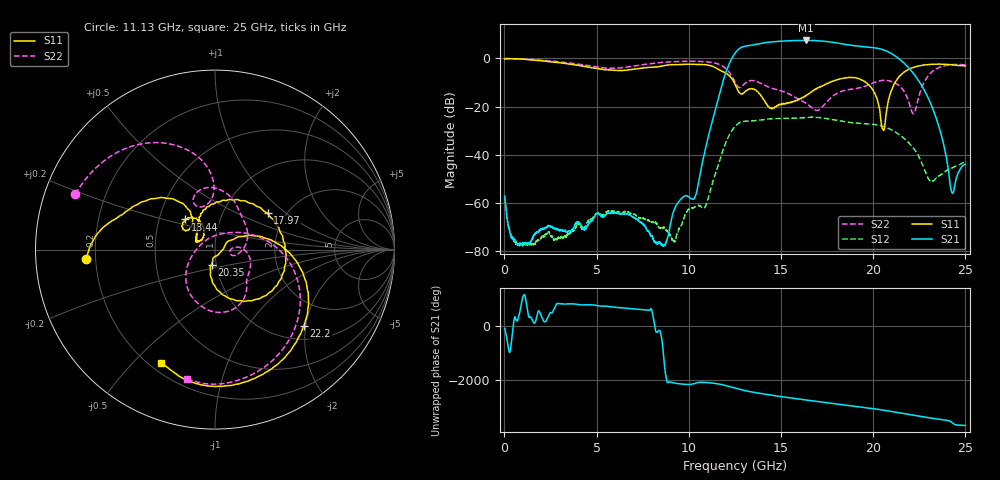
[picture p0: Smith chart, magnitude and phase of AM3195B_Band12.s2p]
!Agilent Technologies,E8364B,MY43040894,A.07.50.67
!Agilent E8364B: A.07.50.67
!Date: Wednesday, July 07, 2021 13:12:42
!Correction: S11(Full 2 Port(1,2))
!S21(Full 2 Port(1,2))
!S12(Full 2 Port(1,2))
!S22(Full 2 Port(1,2))
!S2P File: Measurements: S11, S21, S12, S22:
# Hz S  dB  R 50
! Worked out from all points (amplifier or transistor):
!   8001 points, 10 MHz to 25 GHz, reference 50 ohm
!   highest |S21| = 7.4 dB at 16.37 GHz (marker M1)
!   |S21| within 3 dB of that: 12.82 GHz to 20.05 GHz (7.233 GHz wide, 44 % of centre)
!   unconditionally stable (mu >= 1): start of sweep to end of sweep
!   at 4.174 GHz: K = 1124994.23, MAG = -63.0 dB, |S12| = -70.4 dB
!   at 12.51 GHz: K = 8.23, MAG = 3.0 dB, |S12| = -28.2 dB
!   at 25 GHz: K = 2685.67, MAG = -37.7 dB, |S12| = -43.2 dB
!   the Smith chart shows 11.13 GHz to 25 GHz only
!   S11 on the Smith chart (normalised r, x): 11.13 GHz: 0.16, -0.04; 13.44 GHz: 0.68, +0.24; 17.97 GHz: 1.62, +0.75; 20.35 GHz: 0.95, -0.16; 22.2 GHz: 1.32, -1.95; 25 GHz: 0.25, -0.60
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1e7  -0.26 -1.9  -57.06 -94.1  -57.55 83.0  -0.09 -2.8
1.918611e9  -0.92 -94.0  -71.18 127.3  -74.89 106.2  -0.70 -89.7
4.177082e9  -3.12 165.0  -69.48 53.9  -70.54 61.3  -2.58 164.4
6.594865e9  -4.90 28.7  -64.47 -68.9  -63.62 -58.0  -3.66 7.8
8.341041e9  -3.46 -62.9  -76.27 171.8  -69.73 -159.4  -1.81 -88.2
1.113055e10  -2.87 -175.9  -30.27 43.1  -55.73 -125.9  -1.54 158.3
1.2505e10  -10.63 124.4  2.13 -152.8  -28.21 70.6  -9.85 91.3
1.284861e10  -14.73 139.7  4.54 144.3  -26.37 11.4  -11.78 111.7
1.343588e10  -12.56 134.4  5.52 59.9  -25.89 -71.4  -9.17 95.9
1.408874e10  -17.31 117.3  6.45 -15.2  -25.35 -145.7  -11.03 65.8
1.483532e10  -19.55 156.6  7.06 -93.3  -24.91 137.4  -13.09 40.9
1.5635e10  -18.11 146.7  7.37 -169.7  -24.84 67.0  -15.57 5.8
1.636596e10  -15.33 123.9  7.43 123.6  -24.49 8.2  -18.62 -15.9
1.667208e10  -13.85 114.1  7.42 96.3  -24.38 -17.0  -20.41 -18.0
1.797469e10  -8.96 34.6  6.47 -18.9  -25.64 -120.8  -14.76 -6.6
1.897741e10  -7.98 -29.7  5.25 -103.2  -26.76 162.7  -12.60 -38.7
1.972086e10  -10.76 -71.7  4.73 -168.7  -27.17 100.9  -11.07 -50.9
2.035498e10  -21.36 -103.1  3.98 128.3  -27.82 41.1  -9.31 -69.7
2.083604e10  -17.00 29.2  2.64 75.5  -29.05 -6.8  -9.24 -92.7
2.220112e10  -3.71 -40.6  -6.44 -80.4  -37.43 -144.3  -22.86 111.5
2.426904e10  -2.66 -104.6  -55.63 8.9  -45.46 -62.1  -2.60 -81.3
2.5e10  -3.13 -115.4  -43.97 -100.1  -43.17 -91.7  -2.67 -102.1
